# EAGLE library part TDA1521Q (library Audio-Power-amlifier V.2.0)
2 x 12 W hi-fi audio power amplifier http://www.datasheetcatalog.org/datasheet/philips/TDA1521Q.pdf
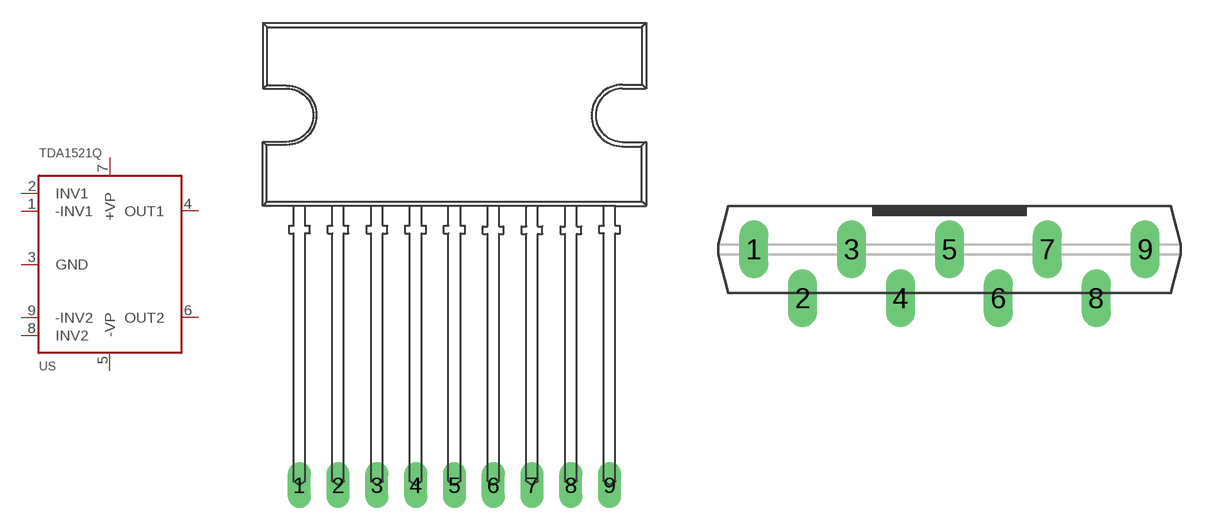
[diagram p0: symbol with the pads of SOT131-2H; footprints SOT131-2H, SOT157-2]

Designator prefix US

## TDA1521QPION  [SOT131-2H]
1  -INV1  in
2  INV1  in
3  GND  in
4  OUT1  in
5  -VP  in
6  OUT2  in
7  +VP  in
8  INV2  in
9  -INV2  in

## TDA1521QSOT157-2  [SOT157-2]
Pads as for SOT131-2H

## Footprint SOT131-2H (pad centres in mm)
drill 1 long: 1 -10.16,0; 2 -7.62,0; 3 -5.08,0; 4 -2.54,0; 5 0,0; 6 2.54,0; 7 5.08,0; 8 7.62,0; 9 10.16,0

## Footprint SOT157-2 (pad centres in mm)
drill 1 long: 1 -10.16,0; 2 -7.62,-2.54; 3 -5.08,0; 4 -2.54,-2.54; 5 0,0; 6 2.54,-2.54; 7 5.08,0; 8 7.62,-2.54; 9 10.16,0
